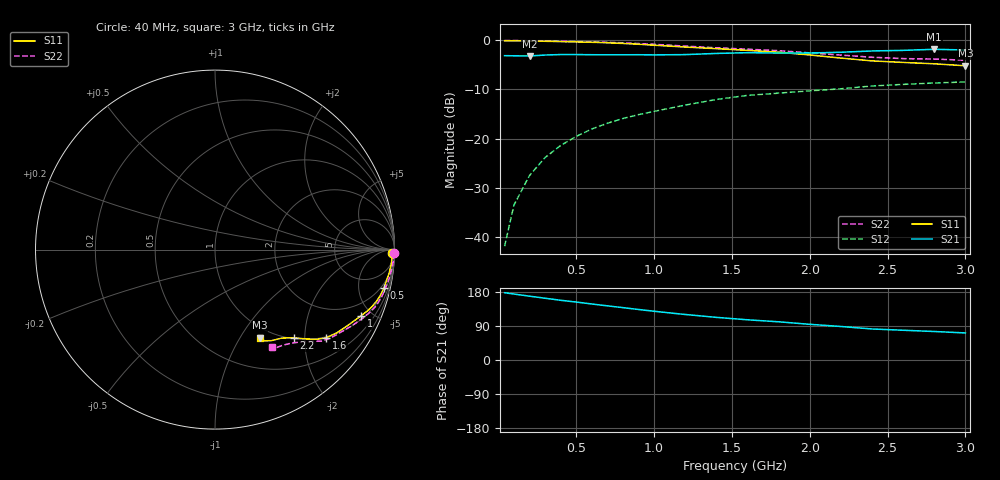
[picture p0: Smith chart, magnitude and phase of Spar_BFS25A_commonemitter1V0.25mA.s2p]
! Filename:  BFS25AB.S2P  Version:  4.0
! NXP part #: BFS25A  Date: Jun 1994
! Bias condition: Vce=1V, Ic=0.25mA
#  MHz  S  MA  R  50
! Freq  S11  S21  S12  S22  !GUM [dB]
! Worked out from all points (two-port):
!   21 points, 40 MHz to 3 GHz, reference 50 ohm
!   highest |S21| = -1.82 dB at 2.8 GHz (marker M1); lowest = -3.2 dB at 200 MHz (marker M2)
!   |S21| within 3 dB of the highest: start of sweep to end of sweep
!   lowest |S11| = -5.2 dB at 3 GHz (marker M3), VSWR 3.45, Z = 43.3 - j61 ohm
!   |S11| at or under -10 dB: nowhere
!   |S22| runs from -4.0 to 0.0 dB; largest |S21 - S12| = 0.71
!   S11 on the Smith chart (normalised r, x): 40 MHz: 52, -82; 500 MHz: 1.38, -8.63; 1 GHz: 1.18, -4.32; 1.6 GHz: 0.97, -2.55; 2.2 GHz: 1.02, -1.77; 3 GHz: 0.87, -1.22
40  0.989 -1.0  0.699 177.5  0.008 89.3  0.998 -1.1
100  0.988 -2.5  0.696 174.1  0.021 86.6  0.997 -2.6
200  0.985 -5.0  0.693 168.4  0.042 83.5  0.993 -5.2
300  0.979 -7.7  0.709 163.0  0.064 80.8  0.987 -7.9
400  0.971 -10.3  0.717 157.6  0.085 78.7  0.98 -10.6
500  0.965 -12.9  0.717 152.9  0.105 76.6  0.972 -13.3
600  0.956 -15.4  0.714 147.8  0.125 74.6  0.965 -15.9
700  0.945 -17.7  0.713 142.9  0.143 72.6  0.955 -18.2
800  0.93 -20.0  0.713 138.2  0.16 70.5  0.944 -20.3
900  0.913 -22.2  0.714 133.3  0.175 68.1  0.928 -22.4
1000  0.893 -24.4  0.711 128.6  0.189 65.7  0.911 -24.5
1200  0.855 -29.3  0.716 120.1  0.219 60.9  0.874 -28.9
1400  0.823 -34.2  0.736 112.5  0.25 57.2  0.84 -33.1
1600  0.791 -38.4  0.749 106.1  0.275 53.6  0.813 -37.1
1800  0.757 -41.3  0.742 100.8  0.29 51.4  0.785 -40.5
2000  0.71 -44.5  0.743 94.2  0.306 48.3  0.746 -43.3
2200  0.66 -48.1  0.757 88.4  0.321 45.6  0.708 -46.5
2400  0.618 -52.9  0.78 81.9  0.343 42.3  0.673 -50.7
2600  0.596 -58.4  0.791 78.5  0.356 39.7  0.652 -54.9
2800  0.577 -61.7  0.811 75.2  0.368 39.2  0.645 -57.8
3000  0.551 -63.1  0.798 71.4  0.377 37.5  0.628 -59.7
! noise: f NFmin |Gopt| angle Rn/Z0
500  1.6  0.935  2  3
1000  1.8  0.92  9  3
2000  2.1  0.796  28  1.6
